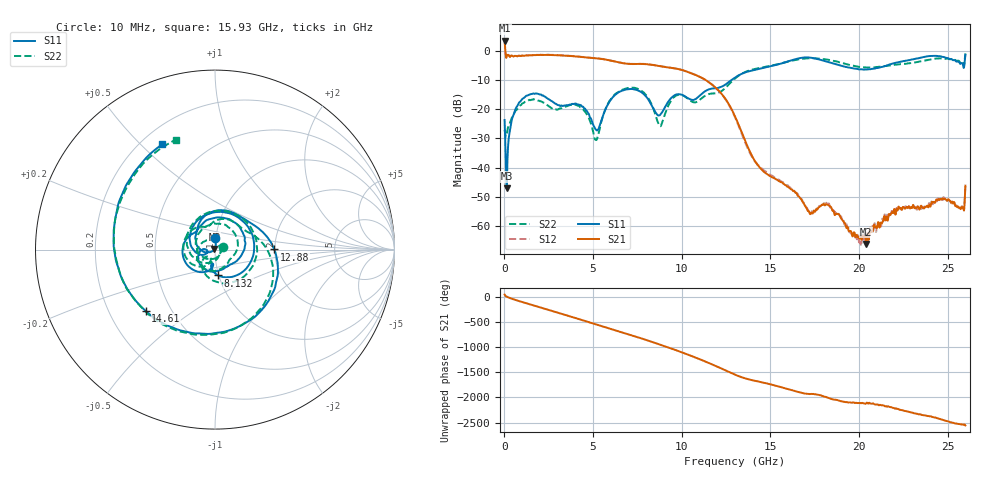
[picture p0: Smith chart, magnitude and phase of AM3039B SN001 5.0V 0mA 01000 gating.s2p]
!Agilent Technologies,E8364B,MY43040894,A.07.50.67
!Agilent E8364B: A.07.50.67
!Date: Tuesday, June 28, 2016 08:05:08
!Correction: S11(Full 2 Port(1,2))
!S21(Full 2 Port(1,2))
!S12(Full 2 Port(1,2))
!S22(Full 2 Port(1,2))
!S2P File: Measurements: S11, S21, S12, S22:
# Hz S  dB  R 50
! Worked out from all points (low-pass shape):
!   1601 points, 10 MHz to 26 GHz, reference 50 ohm
!   highest |S21| = 3.61 dB at 10 MHz (marker M1); lowest = -66.3 dB at 20.41 GHz (marker M2)
!   |S21| within 3 dB of the highest: start of sweep to 44.52 MHz
!   lowest |S11| = -47.2 dB at 123.7 MHz (marker M3), VSWR 1.01, Z = 49.7 + j0.301 ohm
!   |S11| at or under -10 dB: start of sweep to 12.79 GHz
!   |S22| runs from -30.6 to -0.8 dB; largest |S21 - S12| = 0.024
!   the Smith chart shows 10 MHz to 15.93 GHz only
!   S11 on the Smith chart (normalised r, x): 10 MHz: 0.99, +0.13; 8.132 GHz: 0.99, -0.29; 12.88 GHz: 1.99, +0.00; 14.61 GHz: 0.36, -0.33; 15.93 GHz: 0.28, +0.58
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1e7  -23.66 91.2  3.61 40.6  3.67 41.4  -27.06 16.5
1.237062e8  -47.20 136.1  -2.05 1.4  -1.99 1.4  -28.96 -59.1
7.734562e8  -18.31 152.9  -1.61 -83.3  -1.56 -83.0  -19.46 170.0
1.601888e9  -14.63 67.8  -1.37 -171.0  -1.33 -170.9  -16.63 72.7
2.47905e9  -16.44 -12.0  -1.31 97.0  -1.25 97.0  -18.78 -10.5
3.291238e9  -18.81 -57.9  -1.50 11.1  -1.44 11.1  -19.39 -57.9
4.347081e9  -18.84 -139.1  -2.02 -101.9  -1.98 -101.9  -19.52 -166.0
5.792775e9  -18.78 -176.3  -3.00 100.0  -2.95 100.0  -18.60 -150.2
6.783644e9  -13.30 71.1  -4.24 -6.5  -4.20 -6.4  -12.96 67.3
8.131875e9  -16.78 -83.1  -4.55 -156.6  -4.51 -156.3  -16.32 -108.2
8.684162e9  -22.12 -100.9  -5.09 138.0  -5.04 138.5  -24.90 -138.1
1.287505e10  -9.62 0.1  -20.72 -89.4  -20.96 -88.6  -10.13 -7.5
1.3005e10  -9.08 -9.7  -22.43 -108.9  -22.75 -108.3  -9.41 -17.4
1.461313e10  -5.76 -138.5  -41.38 92.5  -40.85 97.5  -5.54 -149.0
1.592888e10  -3.66 116.5  -46.42 -30.2  -46.10 -27.0  -3.73 109.7
1.734208e10  -2.32 -16.5  -55.66 -132.5  -55.00 -133.4  -2.45 -10.3
1.888524e10  -4.87 -151.5  -56.22 93.8  -56.22 92.5  -3.82 -140.9
2.041215e10  -6.33 100.0  -66.30 46.9  -66.07 37.2  -5.65 108.8
2.167916e10  -4.66 15.4  -56.00 -24.1  -56.46 -22.7  -4.99 20.6
2.310861e10  -2.74 -91.9  -53.74 -157.4  -53.97 -151.1  -3.93 -82.6
2.421319e10  -1.62 178.5  -51.80 125.0  -52.08 126.9  -2.66 -166.7
2.6e10  -1.32 -22.0  -46.22 -36.8  -46.25 -41.4  -0.79 6.3
